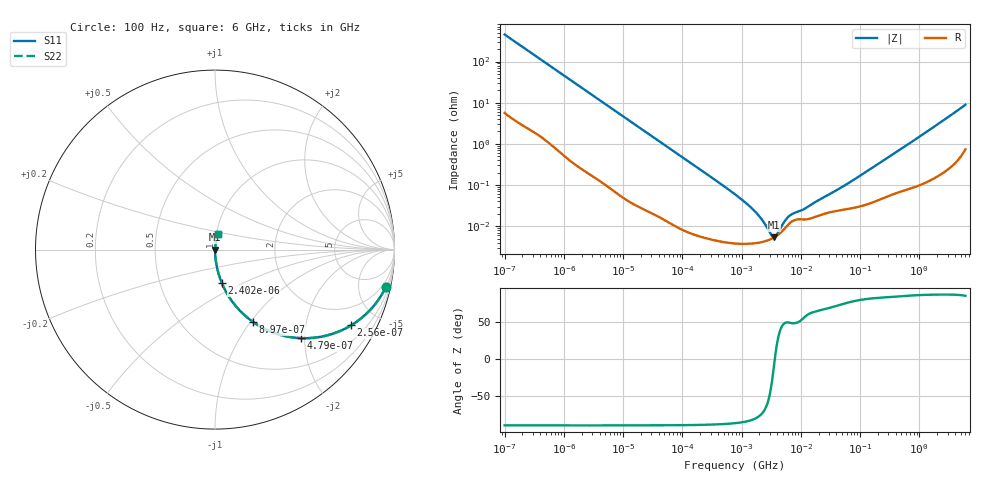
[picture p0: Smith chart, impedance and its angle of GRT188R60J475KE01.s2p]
!Murata Part Number: GRT188R60J475KE01
!These Parameters are Measured in Series Mode Connection
!Data Generated on Jun 19, 2026
!  o--ll--o
!Port1  Port2
!  o------o
!Operation Temp=25[degC], DC Bias Voltage=0[V]
!Freq. Start=100[Hz] Stop=6[GHz] 401[Steps]
# Hz S RI R 50
!Freq.(Hz) S11(Real) S11(Imag) S21(Real) S21(Imag) S12(Real) S12(Imag) S22(Real) S22(Imag)
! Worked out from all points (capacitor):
!   401 points, 100 Hz to 6 GHz, reference 50 ohm
!   read as one part in series: C = 3.5 uF near 109 Hz
!   lowest |Z| = 5.4 mohm at 3.55 MHz (marker M1)
!   series resonance near 3.642 MHz, so ESL is about 550 pH
!   S11 on the Smith chart (normalised r, x): 100 Hz: 1.11, -9.08; 256 Hz: 1.05, -3.57; 479 Hz: 1.03, -1.92; 897 Hz: 1.01, -1.03; 2.402 kHz: 1.00, -0.39; 6 GHz: 1.01, +0.18
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100  0.9514 -0.2089  0.0486 0.2089  0.0486 0.2089  0.9514 -0.2089
164  0.8827 -0.3158  0.1173 0.3158  0.1173 0.3158  0.8827 -0.3158
256  0.7582 -0.4218  0.2418 0.4218  0.2418 0.4218  0.7582 -0.4218
479  0.4795 -0.4931  0.5205 0.4931  0.5205 0.4931  0.4795 -0.4931
897  0.2125 -0.4034  0.7875 0.4034  0.7875 0.4034  0.2125 -0.4034
1283  0.1178 -0.3171  0.8822 0.3171  0.8822 0.3171  0.1178 -0.3171
2008  0.0528 -0.2184  0.9472 0.2184  0.9472 0.2184  0.0528 -0.2184
2402  0.0379 -0.1858  0.9621 0.1858  0.9621 0.1858  0.0379 -0.1858
7358  0.0047 -0.0633  0.9953 0.0633  0.9953 0.0633  0.0047 -0.0633
40335  0.000305 -0.0117  0.9997 0.0117  0.9997 0.0117  0.000305 -0.0117
774597  3.83e-05 -0.000595  1 0.000595  1 0.000595  3.83e-05 -0.000595
1585629  3.82e-05 -0.000247  1 0.000247  1 0.000247  3.82e-05 -0.000247
2594782  4.4e-05 -9.16e-05  1 9.16e-05  1 9.16e-05  4.4e-05 -9.16e-05
3549919  5.36e-05 -6.7e-06  0.9999 6.7e-06  0.9999 6.7e-06  5.36e-05 -6.7e-06
4643984  7.13e-05 6.39e-05  0.9999 -6.39e-05  0.9999 -6.39e-05  7.13e-05 6.39e-05
6644369  0.000122 0.000139  0.9999 -0.000139  0.9999 -0.000139  0.000122 0.000139
1.137099e7  0.000145 0.000216  0.9999 -0.000216  0.9999 -0.000216  0.000145 0.000216
1.555665e7  0.000159 0.000308  0.9998 -0.000308  0.9998 -0.000308  0.000159 0.000308
5.960426e7  0.000261 0.00102  0.9997 -0.00102  0.9997 -0.00102  0.000261 0.00102
3.124326e8  0.000573 0.00487  0.9994 -0.00487  0.9994 -0.00487  0.000573 0.00487
1.873145e9  0.00226 0.0273  0.9977 -0.0273  0.9977 -0.0273  0.00226 0.0273
6e9  0.0149 0.0867  0.9851 -0.0867  0.9851 -0.0867  0.0149 0.0867
